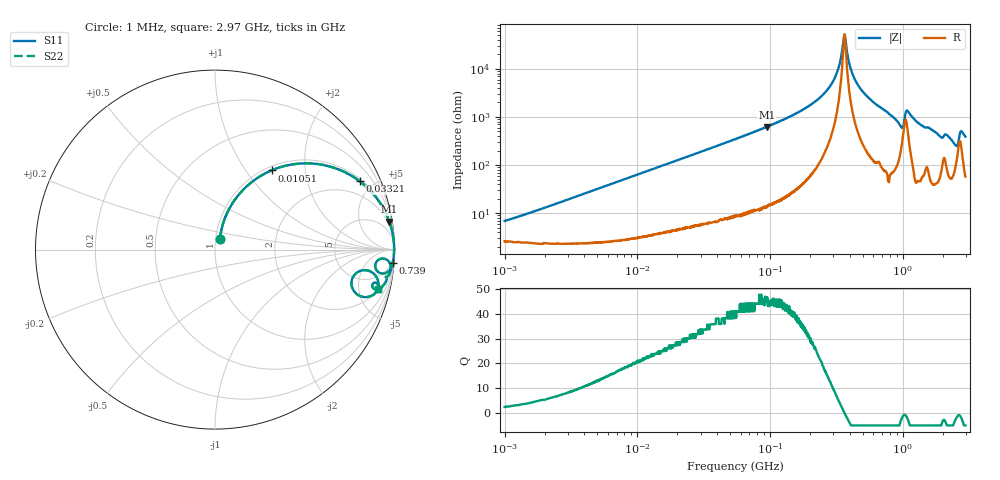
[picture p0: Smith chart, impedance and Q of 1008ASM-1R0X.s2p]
!s-Parameter Generated by FASTRON Sdn. Bhd.
!FASTRON P/N : 1008ASM-1R0X
!Keysight Technologies: E4991B_MY54100416_A.01.15
!Date: Tue Nov 21 09:42:23 2023
!Version  :Rev00  Wed Nov 22 15:06:19 2023
!Data & Calibration Information:
!Freq  S11  S21  S12  S22
!PortZ  Port1:50+j0  Port2:50+j0
!When reading reference impedance value at option line is always used.
! Remarks : This data is being provided solely for informational purposes.
# Hz S dB R 50
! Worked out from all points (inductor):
!   1599 points, 1 MHz to 2.97 GHz, reference 50 ohm
!   read as one part in series: L = 1.02 uH near 1.174 MHz
!   highest Q = 45.1 at 94.5 MHz (marker M1), where L = 1.05 uH
!   self-resonance near 363.1 MHz
!   S11 on the Smith chart (normalised r, x): 1 MHz: 1.05, +0.13; 10.51 MHz: 1.06, +1.33; 33.21 MHz: 1.12, +4.17; 739 MHz: 2, -27; 2.97 GHz: 2.16, -7.73
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1000000  -23.40 64.1  -0.24 -3.6  -0.24 -3.6  -23.40 64.1
3804036  -12.70 71.1  -0.44 -13.3  -0.44 -13.3  -12.70 71.1
1.05052e7  -5.31 54.4  -1.78 -32.8  -1.78 -32.8  -5.31 54.4
1.439846e7  -3.61 46.4  -2.79 -41.2  -2.79 -41.2  -3.61 46.4
3.320783e7  -1.00 25.3  -7.38 -63.0  -7.38 -63.0  -1.00 25.3
5.477226e7  -0.40 16.0  -11.20 -72.6  -11.20 -72.6  -0.40 16.0
9.450168e7  -0.14 9.1  -16.00 -79.7  -16.00 -79.7  -0.14 9.1
2.073156e8  -0.03 3.0  -25.50 -84.9  -25.50 -84.9  -0.03 3.0
3.017325e8  -0.02 1.0  -35.30 -83.0  -35.30 -83.0  -0.02 1.0
3.301716e8  -0.02 0.5  -40.80 -77.9  -40.80 -77.9  -0.02 0.5
3.649251e8  -0.02 -0.0  -54.30 2.5  -54.30 2.5  -0.02 -0.0
4.0536e8  -0.02 -0.6  -40.20 77.5  -40.20 77.5  -0.02 -0.6
4.525341e8  -0.02 -1.1  -34.00 82.6  -34.00 82.6  -0.02 -1.1
7.38967e8  -0.06 -4.2  -22.60 82.6  -22.60 82.6  -0.06 -4.2
7.846996e8  -0.06 -4.8  -21.50 83.0  -21.50 83.0  -0.06 -4.8
9.779672e8  -0.61 -8.1  -16.30 59.7  -16.30 59.7  -0.61 -8.1
1.091779e9  -0.27 -3.9  -22.70 63.7  -22.70 63.7  -0.27 -3.9
1.388188e9  -0.20 -8.4  -16.70 77.1  -16.70 77.1  -0.20 -8.4
2.134733e9  -0.62 -12.2  -13.30 65.4  -13.30 65.4  -0.62 -12.2
2.480502e9  -1.37 -17.8  -9.88 54.3  -9.88 54.3  -1.37 -17.8
2.75535e9  -0.92 -8.8  -15.00 51.1  -15.00 51.1  -0.92 -8.8
2.970126e9  -0.57 -13.7  -12.40 67.8  -12.40 67.8  -0.57 -13.7
